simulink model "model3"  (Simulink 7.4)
settings: Solver=ode23t  StartTime=0.0  StopTime=10.0  RelTol=1e-3
libraries: simulink x1

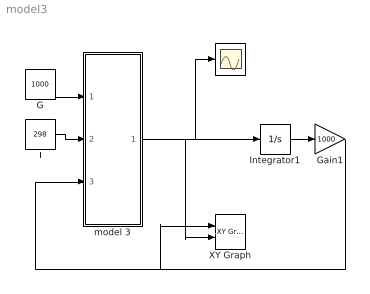
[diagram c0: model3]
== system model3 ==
  G : Constant  Value=1000  OutDataType=sfix(16)  OutScaling=2^0
  Gain1 : Gain  Gain=1000  ParameterDataType=sfix(16)  ParameterScaling=2^0  OutDataType=sfix(16)  OutScaling=2^0
  Integrator1 : Integrator
  T : Constant  Value=298  OutDataType=sfix(16)  OutScaling=2^0
  XY Graph : simulink/Sinks/XY Graph  SystemSampleTime=-1  xmin=0  xmax=50  ymin=0  ymax=5  st=-1
  i : Scope
  model 3 : Subsystem
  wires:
  model 3/1(ipv) -> i/1, Integrator1/1, XY Graph/2
  T/1 -> model 3/2(T)
  G/1 -> model 3/1(G)
  Integrator1/1 -> Gain1/1
  Gain1/1 -> model 3/3(v), XY Graph/1

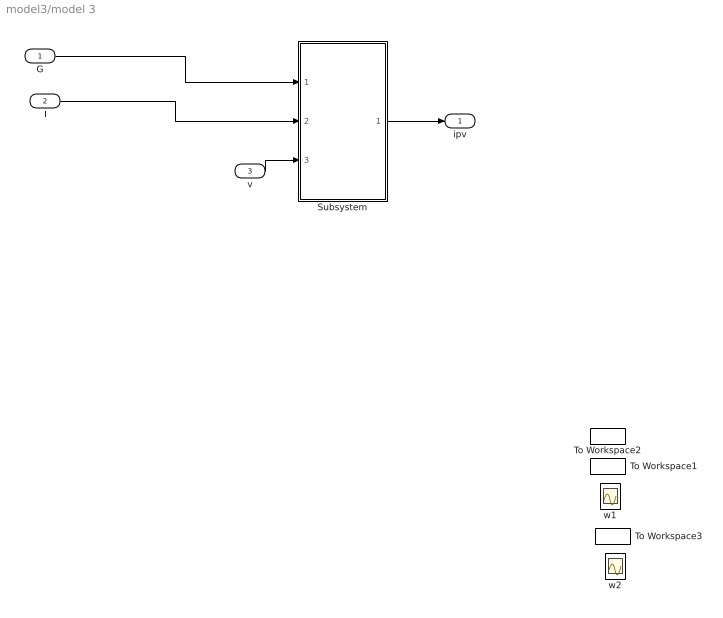
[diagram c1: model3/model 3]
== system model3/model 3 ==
  G : Inport  OutDataType=sfix(16)  OutScaling=2^0
  T : Inport  Port=2  OutDataType=sfix(16)  OutScaling=2^0
  v : Inport  Port=3  OutDataType=sfix(16)  OutScaling=2^0
  Subsystem : Subsystem  mask{Iscst=3.45, Voc=43.5, Im=3.15, Vm=35, alpha=0.014, beta=0.152, K1=9.5652e-5, K2=0.1083, Rs=0.3, Tjref=323, Gsref=1000, Cpv=0.00001}
  To Workspace1 : ToWorkspace  VariableName=i1  SampleTime=-1  SaveFormat=Array
  To Workspace2 : ToWorkspace  VariableName=v1  SampleTime=-1  SaveFormat=Array
  To Workspace3 : ToWorkspace  VariableName=p1  SampleTime=-1  SaveFormat=Array
  w1 : Scope
  w2 : Scope
  ipv : Outport
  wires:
  G/1 -> Subsystem/1(G)
  T/1 -> Subsystem/2(T)
  ? -> To Workspace2/1
  ? -> w1/1
  ? -> To Workspace1/1
  ? -> w2/1
  ? -> To Workspace3/1
  Subsystem/1(ipv) -> ipv/1
  v/1 -> Subsystem/3(v)

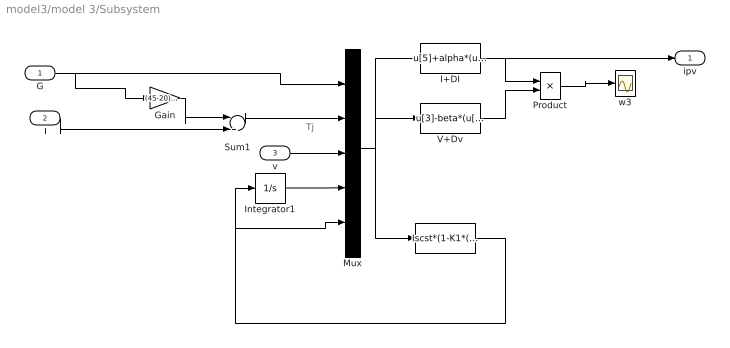
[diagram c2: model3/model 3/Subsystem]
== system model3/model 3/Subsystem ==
  note: Tj
  G : Inport  OutDataType=sfix(16)  OutScaling=2^0
  T : Inport  Port=2  OutDataType=sfix(16)  OutScaling=2^0
  v : Inport  Port=3  OutDataType=sfix(16)  OutScaling=2^0
  Gain : Gain  Gain=(45-20)/800  ParameterDataType=sfix(16)  ParameterScaling=2^0  OutDataType=sfix(16)  OutScaling=2^0
  I : Fcn  Expr=Iscst*(1-K1*(exp(u[3]/(K2*Voc))-1))
  I+DI : Fcn  Expr=u[5]+alpha*(u[1]/Gsref*(u[2]-Tjref))+(u[1]/Gsref-1)*Iscst
  Integrator1 : Integrator
  Mux : Mux  Inputs=5
  Product : Product  OutDataType=sfix(16)  OutScaling=2^0
  Sum1 : Sum  Inputs=|++  OutDataType=sfix(16)  OutScaling=2^0
  V+Dv : Fcn  Expr=u[3]-beta*(u[2]-Tjref)-Rs*alpha*(u[1]/Gsref*(u[2]-Tjref))+(u[1]/Gsref-1)*Iscst
  w3 : Scope
  ipv : Outport
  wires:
  G/1 -> Gain/1, Mux/1
  Mux/1 -> I+DI/1, V+Dv/1, I/1
  I+DI/1 -> Product/1, ipv/1
  V+Dv/1 -> Product/2
  I/1 -> Integrator1/1, Mux/5
  Integrator1/1 -> Mux/4
  Gain/1 -> Sum1/1
  Sum1/1 -> Mux/2
  T/1 -> Sum1/2
  Product/1 -> w3/1
  v/1 -> Mux/3
